// 分隔物料、输送物料的系统
FUNCTION_BLOCK FB_SeparatingModule EXTENDS FB_Subsystem_Root
VAR_INPUT
	// =============== Control the state and mode of machine ========================
	bExecute					: BOOL;							// 如果为TRUE，则该系统进入运行状态
	bSemiStart					: BOOL;							// 如果为TRUE，则将改系统切换至半自动状态
	
	// =============== Information about number of boxes being sorted ===============
	nBoxesOnTheWay				: INT;							// 当前输送皮带上的物料数量
	
	// =============== Cylinders buttons ============================================
	bButtonClampToWorkIn   AT%I*: BOOL;							// 将正位气缸移动到目标位置的按钮
	bButtonClampToBaseIn   		: BOOL;							// 将正位气缸移动到基始位置的按钮
	bButtonBarrierToWorkIn AT%I*: BOOL;							// 将栏杆气缸移动到基始位置的按钮
	bButtonBarrierToBaseIn 		: BOOL;							// 将栏杆气缸移动到基始位置的按钮
END_VAR
VAR_OUTPUT
	// =============== Process information ==========================================
	bSeparated					: BOOL;							// 如果为TRUE，则分割物料完成

	// =============== For movement simulation on visualization =====================
	bClampToWork				: BOOL;							// 如果为TRUE，则正位气缸往目标位置移动的信号为TRUE
	bBarrierToWork				: BOOL;							// 如果为TRUE，则栏杆气缸往目标位置移动的信号为TRUE
		
	// =============== Error variables ==============================================
	bClampError					: BOOL;							// 如果为TRUE，则正位气缸发生报错
	sClampErrorMsg				: STRING;						// 正位气缸的报错信息
	bBarrierError				: BOOL;							// 如果为TRUE，则栏杆气缸发生报错
	sBarrierErrorMsg			: STRING;						// 栏杆气缸的报错信息
	
	// =============== Temperature recordings =======================================
	aClampTemps					: ARRAY[1..100] OF LREAL;		// 正位气缸记录的温度数据
	aBarrierTemps				: ARRAY[1..100] OF LREAL;		// 栏杆气缸记录的温度数据
	
	// =============== Button return signals ========================================
	bButtonClampToWorkOut		: BOOL;							// 将正位气缸移动到目标位置的按钮信号经过信号处理功能块的输出
	bButtonClampToBaseOut		: BOOL;							// 将正位气缸移动到基始位置的按钮信号经过信号处理功能块的输出
	bButtonBarrierToWorkOut		: BOOL;							// 将栏杆气缸移动到目标位置的按钮信号经过信号处理功能块的输出
	bButtonBarrierToBaseOut		: BOOL;							// 将栏杆气缸移动到基始位置的按钮信号经过信号处理功能块的输出
END_VAR

VAR
	// =============== Function block instance of sensor ============================
	fbSensor					: FB_SignalHandling;			// 信号处理功能块
	
	// =============== Function block instances for clamp cylinder ==================
	fbClamp						: FB_Cylinder;					// 正位气缸对象
	
	// =============== Function block instances for barrier cylinder ================
	fbBarrier					: FB_Cylinder;					// 栏杆气缸对象
		
	// =============== Cylinder parameters for clamp and barrier ====================
	tTimeOutClamp				: TIME;							// 判定正位气缸为超时的设定时间
	tTimeOutBarrier				: TIME;							// 判定栏杆气缸为超时的设定时间
	tRecordIntervalClamp		: TIME;							// 记录正位气缸温度的时间
	tRecordIntervalBarrier		: TIME;							// 记录栏杆气缸温度的时间
	tBarrierAtWork				: TIME;							// 栏杆气缸打开的时间（目标位置）
	
	// =============== Manual cylinder control ======================================
	fbButtonClampToWork			: FB_SignalHandling;			// 处理正位气缸移动到目标位置的按钮信号功能块
	fbButtonClampToBase			: FB_SignalHandling;			// 处理正位气缸移动到基始位置的按钮信号功能块
	fbButtonBarrierToWork		: FB_SignalHandling;			// 处理栏杆气缸移动到目标位置的按钮信号功能块
	fbButtonBarrierToBase		: FB_SignalHandling;			// 处理栏杆气缸移动到基始位置的按钮信号功能块
	
	// =============== Common variables ==============================================
	fbTimerBarrierAtWork		: TON;							// 处理栏杆气缸打开延时的TON功能块
	eStateAuto					: E_StateSeparatingAuto;		// 自动流程的CASE变量
	eStateSemiAuto				: E_StateSeparatingAuto;		// 半自动流程的CASE变量
	fbTriggerSemiHalt           : R_TRIG;						// 半自动暂停信号的上升沿功能块
	
	BoxUndertheCylinderPosition	: BOOL;							// 如果为TRUE，则物料到达指定气缸的正下方（输送皮带暂停输送的标志位）
	rtBoxUndertheCylinderPosition: R_TRIG;						// 物料到达指定气缸的正下方的上升沿功能块
	
	CylinderWorkDone			: BOOL;							// 如果为TRUE，指定气缸到达目标位置（输送皮带回复输送的标志位）
	rtCylinderWorkDone			: R_TRIG;						// 物料到达指定气缸的正下方的上升沿功能块
	
	HaltRequestTemp				: BOOL;							// 临时暂停请求，用于确保在HaltDone之前继续执行暂停
END_VAR

// =========================================================
;
// =========================================================

METHOD Automatic
VAR_INPUT
END_VAR
// =========================================================
// 检测物料在气缸正下方、分拣系统气缸到目标位	
	rtBoxUndertheCylinderPosition(CLK:= BoxUndertheCylinderPosition);
	rtCylinderWorkDone			 (CLK:= CylinderWorkDone);
	
// 栏杆气缸延迟的TON功能块
	fbTimerBarrierAtWork		 (PT := tBarrierAtWork);

// =========================================================
// 输送皮带控制

// 检查 bHaltRequest（停机请求）是否为真，并且 HaltRequestTemp（临时停机请求）为假。如果条件成立，调用Halt方法。
    IF bHaltRequest THEN
		Halt(bHalt := TRUE);
			
// 其他情况下，轴一直转			
	ELSE		
		fbAxis.MoveFw();
		Halt(bHalt := FALSE);
	END_IF

// =========================================================
// 分割物料的过程
	
	CASE eStateAuto OF
		
		// ==========================初始化===============================
		E_StateSeparatingAuto.Init:
		
				// 确保栏杆气缸回到基始位
				fbBarrier.MoveToBase();
				
				// 栏杆气缸回到基始位完成之后且bExecute为TRUE之后，进入Start步
				IF fbBarrier.bState_AtBasePos AND bExecute THEN
					eStateAuto := E_StateSeparatingAuto.Start;
				END_IF
			
		// =========================================================
		E_StateSeparatingAuto.Start:
		
				// 如果输送带上的传感器检测到物料、且输送皮带在移动，进入到CloseClamp步
				IF fbSensor.bOut AND fbAxis.bMoves THEN
					eStateAuto := E_StateSeparatingAuto.CloseClamp;
				
				// 如果正位气缸没有到达目标位置、让气缸移动到目标位置，确保待输送的物料能移动到栏杆前
				ELSIF NOT fbClamp.bState_AtWorkPos THEN
					fbClamp.MoveToWork();
				END_IF
			
		// =========================================================
		E_StateSeparatingAuto.CloseClamp:
				
				// 检测到栏杆前已经存在物料了，将正位气缸移动到基始位置，固定后续的物料
				fbClamp.MoveToBase();
				
				// 如果正位气缸到达基始位置，也就是固定好物料之后，则bSeparated为TRUE，判定为物料分割完成，进入到OpenBarrier步
				IF fbClamp.bState_AtBasePos THEN
					bSeparated 	:= TRUE;
					eStateAuto 	:= E_StateSeparatingAuto.OpenBarrier;
				END_IF
			
		// =========================================================
		E_StateSeparatingAuto.OpenBarrier:
				
				// 将栏杆气缸移动到目标位，确保物料能够被运出
				fbBarrier.MoveToWork();			
				
				// 如果正位气缸到达目标位置、则将TON的IN置为TRUE
				IF fbBarrier.bState_AtWorkPos THEN
					fbTimerBarrierAtWork.IN := TRUE;
				END_IF
				
				// 到达设定时间之后，复位计时器，进入到CloseBarrier步
				IF fbTimerBarrierAtWork.Q THEN
					fbTimerBarrierAtWork.IN := FALSE;
					eStateAuto := E_StateSeparatingAuto.CloseBarrier;
				END_IF
			
		// =========================================================
		E_StateSeparatingAuto.CloseBarrier:
		
				// 将栏杆气缸移动到基始位置
				fbBarrier.MoveToBase();
				
				// 如果栏杆气缸到达基始位置，进入到OpenClamp步
				IF fbBarrier.bState_AtBasePos THEN
					bSeparated 	:= FALSE;
					eStateAuto	:= E_StateSeparatingAuto.OpenClamp;
				END_IF
			
		// =========================================================
		E_StateSeparatingAuto.OpenClamp:		
				// 将正位气缸移动到目标位置，让下一批物料推进
				fbClamp.MoveToWork();
				
				// 如果正位气缸到达目标位置，回到Init步
				IF fbClamp.bState_AtWorkPos THEN
					eStateAuto := E_StateSeparatingAuto.Init;
				END_IF
	END_CASE

// =========================================================
END_METHOD

PROPERTY bState_BarrierAtBasePos : BOOL
GET
bState_BarrierAtBasePos := fbBarrier.bState_AtBasePos;
END_GET
END_PROPERTY

PROPERTY bState_BarrierAtWorkPos : BOOL
GET
bState_BarrierAtWorkPos := fbBarrier.bState_AtWorkPos;
END_GET
END_PROPERTY

PROPERTY bState_ClampAtBasePos : BOOL
GET
bState_ClampAtBasePos := fbClamp.bState_AtBasePos;
END_GET
END_PROPERTY

PROPERTY bState_ClampAtWorkPos : BOOL
GET
bState_ClampAtWorkPos := fbClamp.bState_AtWorkPos;
END_GET
END_PROPERTY

METHOD CylinderOptions
VAR_INPUT
	bClampDiag			: BOOL;		// If true the clamp cylinder has diagnosis functionality
	bClampTemp			: BOOL;		// If true the clamp cylinder has temperature functionality
	bClampRecord		: BOOL;		// If true the clamp cylinder has recording functionality
	bBarrierDiag		: BOOL;		// If true the barrier cylinder has diagnosis functionality
	bBarrierTemp		: BOOL;		// If true the barrier cylinder has temperature functionality
	bBarrierRecord		: BOOL;		// If true the barrier cylinder has recording functionality
END_VAR
// =========================================================
// Selecting clamp cylinder

	// Checking variables to enable/disable diagnosis and temperature mode
	IF bClampDiag THEN
		IF bClampTemp THEN
			// ============== FB with diagnosis and temperature mode ==============
			bClampError 	:= fbClampTempDiag.bError;								// Assigning output variable of chosen FB to local output variable
			sClampErrorMsg 	:= fbClampTempDiag.sErrorMsg;
			fbClamp 		:= fbClampTempDiag;										// Assigning chosen FB instance to interface instance
		
		ELSE
			// ============== FB with diagnosis and without temperature mode ==============
			fbClampDiag.tTimeOut 	:= tTimeOutClamp;								// Setting special data for selected FB
			bClampError 			:= fbClampDiag.bError;							// Assigning output variable of chosen FB to local output variable	
			sClampErrorMsg 			:= fbClampDiag.sErrorMsg;
			fbClamp 				:= fbClampDiag;									// Assigning chosen FB instance to interface instance
		END_IF
	ELSE
		bClampError 	:= FALSE;
		sClampErrorMsg 	:= '';
		
		IF bClampTemp THEN
			IF bClampRecord THEN
				// ============== FB without diagnosis and with temperature recording ==============
				fbClampTempRecord.tIntervalTime	:= tRecordIntervalClamp;			// Time of record interval
				fbClampTempRecord.bRecordStart	:= bComprAirEnabledLocal;			// Recording if compressed air is set
				
				fbClampTempRecord.Record();											// Calling method of function block FB_CylinderTempRecord
				
				aClampTemps 	:= fbClampTempRecord.aTemps;						// Saving output variable
				fbClamp 		:= fbClampTempRecord;								// Assigning chosen FB instance to interface instance
			ELSE
				// ============== FB without diagnosis and with temperature mode, but without recording ==============
				fbClamp 		:= fbClampTemp;										// Assigning chosen FB instance to interface instance
			END_IF
		ELSE
			// ============== FB without diagnosis and without temperature mode ==============
			fbClamp := fbClamp;														// Assigning chosen FB instance to interface instance		
		END_IF	
	END_IF
									
// =========================================================
// Selecting barrier cylinder

	// Checking variables to enable/disable diagnosis and temperature mode
	IF bBarrierDiag THEN
		IF bBarrierTemp THEN
			// ============== FB with diagnosis and temperature mode ==============
			bBarrierError 		:= fbBarrierTempDiag.bError;						// Assigning output variable of chosen FB to local output variable
			sBarrierErrorMsg 	:= fbBarrierTempDiag.sErrorMsg;
			fbCylinder 			:= fbBarrierTempDiag;								// Assigning chosen FB instance to interface instance
		
		ELSE
			// ============== FB with diagnosis and without temperature mode ==============
			fbBarrierDiag.tTimeOut	:= tTimeOutBarrier;								// Setting special data for selected FB
			bBarrierError 			:= fbBarrierDiag.bError;						// Assigning output variable of chosen FB to local output variable
			sBarrierErrorMsg 		:= fbBarrierDiag.sErrorMsg;
			fbCylinder 				:= fbBarrierDiag;								// Assigning chosen FB instance to interface instance
		END_IF
	ELSE
		bBarrierError := FALSE;
		sBarrierErrorMsg := '';
		
		IF bBarrierTemp THEN
			IF bBarrierRecord THEN
				// ============== FB without diagnosis and with temperature recording ==============
				fbBarrierTempRecord.tIntervalTime 	:= tRecordIntervalBarrier;		// Time of record interval
				fbBarrierTempRecord.bRecordStart 	:= bComprAirEnabledLocal;		// Recording if compressed air is set
				
				fbBarrierTempRecord.Record();										// Calling method of function block FB_CylinderTempRecord
				
				aBarrierTemps 	:= fbBarrierTempRecord.aTemps;						// Saving output variable
				fbCylinder 		:= fbBarrierTempRecord;								// Assigning chosen FB instance to interface instance
			ELSE
				// ============== FB without diagnosis and with temperature mode, but without recording ==============
				fbCylinder 		:= fbBarrierTemp; 									// Assigning chosen FB instance to interface instance
			END_IF
		ELSE
			// ============== FB without diagnosis and without temperature mode ==============
			fbCylinder := fbBarrier;													// Assigning chosen FB instance to interface instance				
		END_IF	
	END_IF
									
// =========================================================
END_METHOD

METHOD Enable
VAR_INPUT
	bComprAirEnabled		: BOOL;			// Enable of compressed air
	bAxisEnable				: BOOL;			// Enable of axis
	bSensorEnable			: BOOL;			// Enable of sensor
	bManualAxisEnable		: BOOL;			// Enable of manual axis control
END_VAR
// =========================================================
// Calling method Enable of base class FB_Module via 'SUPER^.'
		
	SUPER^.Enable(	bComprAirEnabled	:= bComprAirEnabled,
					bAxisEnable			:= bAxisEnable,
					bSensorEnable		:= bSensorEnable,
					bManualAxisEnable	:= bManualAxisEnable);

// =========================================================
// Sensor control
		
	fbSensor.Enable(bEnable := bSensorEnable);

// =========================================================
// Cylinder control (accessing property of FB via interfaces intances)
	
	// Clamp cylinder
	fbButtonClampToWork.Enable(bEnable := bManualCylinderEnable );		
	fbButtonClampToBase.Enable(bEnable := bManualCylinderEnable );
	
	
	// Barrier cylinder
	fbButtonBarrierToWork.Enable(bEnable := bManualCylinderEnable );
	fbButtonBarrierToBase.Enable(bEnable := bManualCylinderEnable );
	

// =========================================================
END_METHOD

METHOD InputOutput
VAR_INPUT
END_VAR
// =========================================================
// Calling method SetOutput of base class FB_Module via 'SUPER^.'
		
	SUPER^.InputOutput();						

// =========================================================
// Sensor
		
	fbSensor.SetOutput();

// =========================================================
// Cylinder buttons
		
	fbButtonClampToWork.SetOutput();
	fbButtonClampToBase.SetOutput();
	fbButtonBarrierToWork.SetOutput();
	fbButtonBarrierToBase.SetOutput();

// =========================================================
// Output variables for cylinders
	
	// Accessing properties of selected FB via interface instances
	bClampToWork 	:= fbClamp.bState_MoveToWork;
	bBarrierToWork 	:= fbBarrier.bState_MoveToWork;

// =========================================================
// Buttons
    bButtonBarrierToBaseIn:= NOT bButtonBarrierToWorkIn;
	bButtonClampToBaseIn  := NOT bButtonClampToWorkIn;

    fbButtonBarrierToBase( bInput:= bButtonBarrierToBaseIn AND NOT bButtonBarrierToWorkIn, bOut=> bButtonBarrierToBaseOut );
    fbButtonBarrierToWork( bInput:= bButtonBarrierToWorkIn AND NOT bButtonBarrierToBaseIn, bOut=> bButtonBarrierToWorkOut );
    fbButtonClampToBase  ( bInput:= bButtonClampToBaseIn   AND NOT bButtonClampToWorkIn  , bOut=> bButtonClampToBaseOut   );
    fbButtonClampToWork  ( bInput:= bButtonClampToWorkIn   AND NOT bButtonClampToBaseIn  , bOut=> bButtonClampToWorkOut   );

// =========================================================
END_METHOD

METHOD Maintenance
VAR_INPUT
END_VAR
// =========================================================
// Calling own method Manual of this class FB_SeparatingModule via 'THIS^.'
		
	THIS^.Manual();				

// =========================================================
END_METHOD

METHOD Manual
VAR_INPUT
END_VAR
// =========================================================
// Calling method Manual of base class FB_Module via 'SUPER^.'
		
	SUPER^.Manual();							

// =========================================================
// Manual cylinder control (Calling methods of FBs via interface instances)
	
	// Clamp cylinder to work position
	IF fbButtonClampToWork.bOut THEN
		fbClamp.MoveToWork();
	// Clamp cylinder to base position
	ELSIF fbButtonClampToBase.bOut THEN
		fbClamp.MoveToBase();
	END_IF
	
	// Barrier cylinder to work position
	IF fbButtonBarrierToWork.bOut THEN
		fbBarrier.MoveToWork();
	// Barrier cylinder to base position
	ELSIF fbButtonBarrierToBase.bOut THEN
		fbBarrier.MoveToBase();
	END_IF

// =========================================================
END_METHOD

PROPERTY P_BoxUndertheCylinderPosition : BOOL
GET
P_BoxUndertheCylinderPosition	:= BoxUndertheCylinderPosition;
END_GET
SET
BoxUndertheCylinderPosition	:= P_BoxUndertheCylinderPosition;
END_SET
END_PROPERTY

PROPERTY P_CylinderWorkDone : BOOL
GET
P_CylinderWorkDone	:= CylinderWorkDone;
END_GET
SET
CylinderWorkDone	:= P_CylinderWorkDone;
END_SET
END_PROPERTY

METHOD Reset
VAR_INPUT
	bReset		: BOOL;				// True if machine is in state RESETTING
END_VAR
// =========================================================
// Calling method Reset of base class FB_Module via 'SUPER^.'
		
	SUPER^.Reset(bReset := bReset);

// =========================================================
// Resetting cylinder and axis
	
	IF fbTriggerResetStart.Q THEN
		bSeparated := FALSE;
		HaltRequestTemp	:= FALSE;
		fbTimerBarrierAtWork(IN := FALSE);
		
		// Calling methods of FBs via interface instances
		fbClamp.Reset();
		fbBarrier.Reset();
	END_IF

// =========================================================
END_METHOD

METHOD PROTECTED ResetState
VAR_INPUT
END_VAR
// =========================================================

eStateAuto 		:= E_StateSeparatingAuto.Init;
eStateSemiAuto	:= E_StateSeparatingAuto.Init;
//eStateAxisAuto	:= E_StateSeparatingAxisAuto.Moving;

// =========================================================
END_METHOD

METHOD Semiautomatic
VAR_INPUT
END_VAR
// =========================================================
// 检测物料在气缸正下方、分拣系统气缸到目标位	
	rtBoxUndertheCylinderPosition(CLK:= BoxUndertheCylinderPosition);
	rtCylinderWorkDone			 (CLK:= CylinderWorkDone);
	fbTimerBarrierAtWork		 (PT := tBarrierAtWork);

// =========================================================
// 输送皮带控制

// 检查 在运输过程当中物料的数量是否为0，并且流程步在初始化阶段。如果条件成立，调用Halt方法。    
    IF (nBoxesOnTheWay = 0) AND (eStateSemiAuto = E_StateSeparatingAuto.Init) THEN
		Halt(bHalt := TRUE);
		
// 检测到物料到达气缸正下方的上升沿，那么将HaltRequestTemp置为TRUE，并调用Halt方法
	ELSIF rtBoxUndertheCylinderPosition.Q THEN 
		HaltRequestTemp	:= TRUE;
		Halt(bHalt := TRUE);
		
// 如果停止没有完成，且HaltRequestTemp为TRUE，依然执行Halt方法，确保上一步执行完成
	ELSIF (NOT bHaltDone) AND HaltRequestTemp THEN
			Halt(bHalt := TRUE);
			IF bHaltDone THEN
				 HaltRequestTemp	:= FALSE;
			END_IF
			
// 其他情况下，轴一直转	
	ELSE	
		fbAxis.MoveFw();
		Halt(bHalt := FALSE);
	END_IF


// =========================================================
// 分割物料的过程
	
	CASE eStateSemiAuto OF
		// =========================================================
		E_StateSeparatingAuto.Init:
		
				// 确保栏杆气缸回到基始位
				fbBarrier.MoveToBase();
				
				// 栏杆气缸回到基始位完成之后且bExecute和bSemiStart（每一次半自动模式下按下的启动信号）都为TRUE之后，进入Start步
				IF fbBarrier.bState_AtBasePos AND bExecute AND bSemiStart THEN
					eStateSemiAuto := E_StateSeparatingAuto.Start;
				END_IF
			
		// =========================================================
		E_StateSeparatingAuto.Start:
		
				// 如果输送带上的传感器检测到物料、且输送皮带在移动，进入到CloseClamp步
				IF fbSensor.bOut THEN
					eStateSemiAuto := E_StateSeparatingAuto.CloseClamp;
					
				// 如果正位气缸没有到达目标位置、让气缸移动到目标位置，确保待输送的物料能移动到栏杆前	
				ELSIF NOT fbClamp.bState_AtWorkPos THEN
						fbClamp.MoveToWork();
				END_IF

			
		// =========================================================
		E_StateSeparatingAuto.CloseClamp:
		
				// 检测到栏杆前已经存在物料了，将正位气缸移动到基始位置，固定后续的物料
				fbClamp.MoveToBase();
				
				// 如果正位气缸到达基始位置，也就是固定好物料之后，则bSeparated为TRUE，判定为物料分割完成，进入到OpenBarrier步
				IF fbClamp.bState_AtBasePos THEN
					bSeparated 		:= TRUE;
					eStateSemiAuto 	:= E_StateSeparatingAuto.OpenBarrier;
				END_IF
			
		// =========================================================
		E_StateSeparatingAuto.OpenBarrier:
		
				// 将栏杆气缸移动到目标位，确保物料能够被运出
				fbBarrier.MoveToWork();
				
				// 如果正位气缸到达目标位置、则将TON的IN置为TRUE
				IF fbBarrier.bState_AtWorkPos THEN
					fbTimerBarrierAtWork.IN := TRUE ;
				END_IF
				
				// 到达设定时间之后，复位计时器，进入到CloseBarrier步
				IF fbTimerBarrierAtWork.Q THEN
					fbTimerBarrierAtWork.IN := FALSE ;
					eStateSemiAuto := E_StateSeparatingAuto.CloseBarrier;
				END_IF
			
		// =========================================================
		E_StateSeparatingAuto.CloseBarrier:
		
				/// 将栏杆气缸移动到基始位置
				fbBarrier.MoveToBase();
				
				// 如果栏杆气缸到达基始位置，进入到OpenClamp步
				IF fbBarrier.bState_AtBasePos THEN
					bSeparated 		:= FALSE;
					eStateSemiAuto 	:= E_StateSeparatingAuto.OpenClamp;
				END_IF
			
		// =========================================================
		E_StateSeparatingAuto.OpenClamp:
		
				// 将正位气缸移动到目标位置，让下一批物料推进
				fbClamp.MoveToWork();
				
				// 如果正位气缸到达目标位置，回到Init步
				IF fbClamp.bState_AtWorkPos THEN
					eStateSemiAuto := E_StateSeparatingAuto.Init;
				END_IF
	END_CASE

// =========================================================
END_METHOD

PROPERTY tBarrierAtWorkPos : TIME
GET
tBarrierAtWorkPos := tBarrierAtWork;
END_GET
SET
tBarrierAtWork := tBarrierAtWorkPos;
END_SET
END_PROPERTY

PROPERTY tRecordIntervalOfBarrier : TIME
GET
tRecordIntervalOfBarrier := tRecordIntervalBarrier;
END_GET
SET
tRecordIntervalBarrier := tRecordIntervalOfBarrier;
END_SET
END_PROPERTY

PROPERTY tRecordIntervalOfClamp : TIME
GET
tRecordIntervalOfClamp := tRecordIntervalClamp;
END_GET
SET
tRecordIntervalClamp := tRecordIntervalOfClamp;
END_SET
END_PROPERTY

PROPERTY tTimeOutOfBarrier : TIME
GET
tTimeOutOfBarrier := tTimeOutBarrier;
END_GET
SET
tTimeOutBarrier := tTimeOutOfBarrier;
END_SET
END_PROPERTY

PROPERTY tTimeOutOfClamp : TIME
GET
tTimeOutOfClamp := tTimeOutClamp;
END_GET
SET
tTimeOutClamp := tTimeOutOfClamp;
END_SET
END_PROPERTY

END_FUNCTION_BLOCK
